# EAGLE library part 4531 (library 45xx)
12-bit PARITY TREE
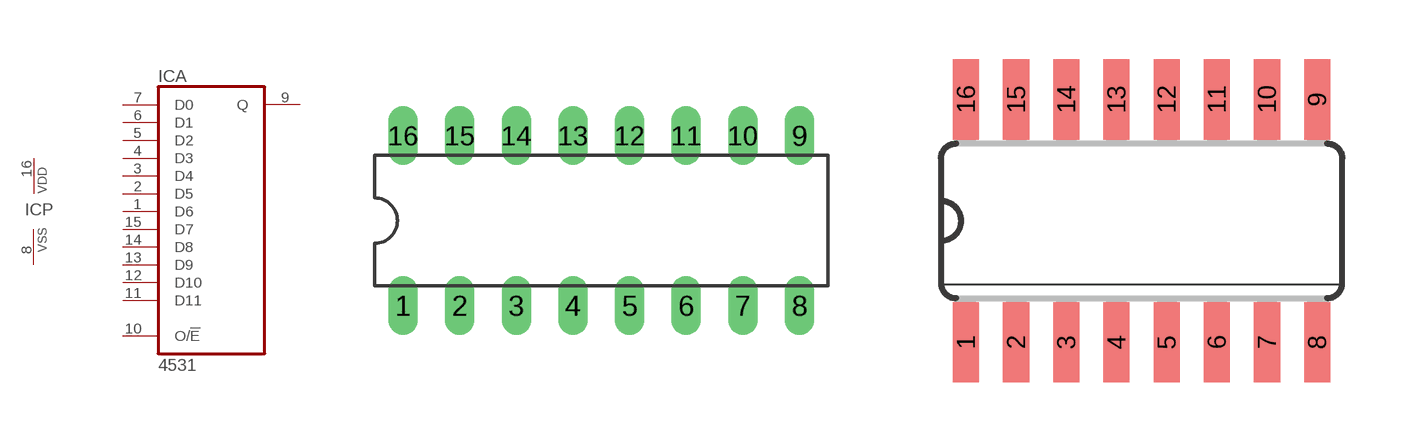
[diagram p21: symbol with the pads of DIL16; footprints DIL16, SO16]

Designator prefix IC; gates A=4531 P=PWRN

## 4531N  [DIL16]
1  A:D6  in
2  A:D5  in
3  A:D4  in
4  A:D3  in
5  A:D2  in
6  A:D1  in
7  A:D0  in
8  P:VSS  pwr
9  A:Q  out
10  A:O/!E  in
11  A:D11  in
12  A:D10  in
13  A:D9  in
14  A:D8  in
15  A:D7  in
16  P:VDD  pwr

## 4531D  [SO16]
Pads as for DIL16

## Footprint DIL16 (pad centres in mm)
Dual In Line Package
drill 0.813 long: 1 -8.89,-3.81; 2 -6.35,-3.81; 3 -3.81,-3.81; 4 -1.27,-3.81; 5 1.27,-3.81; 6 3.81,-3.81; 7 6.35,-3.81; 8 8.89,-3.81; 9 8.89,3.81; 10 6.35,3.81; 11 3.81,3.81; 12 1.27,3.81; 13 -1.27,3.81; 14 -3.81,3.81; 15 -6.35,3.81; 16 -8.89,3.81

## Footprint SO16 (pad centres in mm)
Small Outline package 150 mil
smd 0.66 x 2.032: 1 -4.445,-3.073; 2 -3.175,-3.073; 3 -1.905,-3.073; 4 -0.635,-3.073; 5 0.635,-3.073; 6 1.905,-3.073; 7 3.175,-3.073; 8 4.445,-3.073; 9 4.445,3.073; 10 3.175,3.073; 11 1.905,3.073; 12 0.635,3.073; 13 -0.635,3.073; 14 -1.905,3.073; 15 -3.175,3.073; 16 -4.445,3.073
